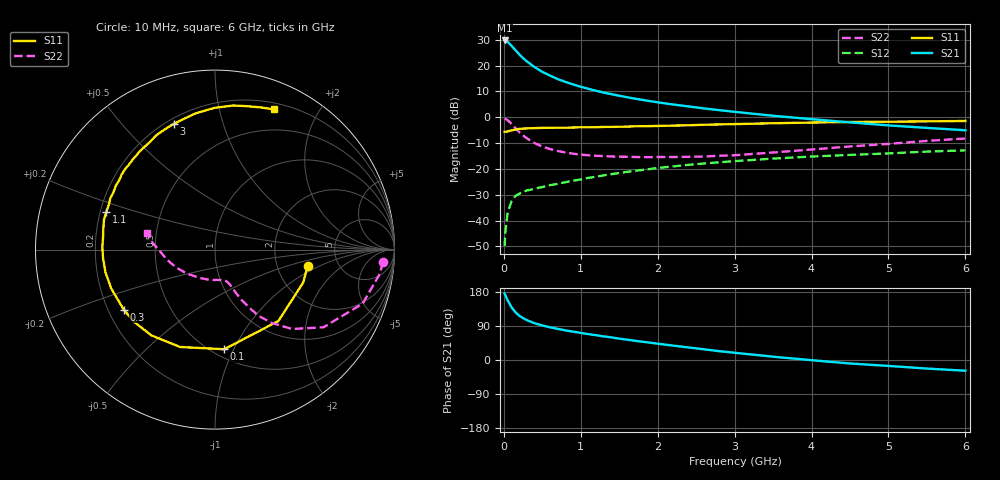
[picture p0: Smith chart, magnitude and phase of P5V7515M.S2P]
! SIEMENS Small Signal Semiconductors
! BFP183
! Si NPN RF Bipolar Junction Transistor in SOT143
! VCE = 0.75 V  IC = 15 mA
! Common Emitter S-Parameters:  March  1996
# GHz  S  MA  R  50
!  f  S11  S21  S12  S22
! GHz  MAG  ANG  MAG  ANG  MAG  ANG  MAG  ANG
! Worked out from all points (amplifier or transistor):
!   36 points, 10 MHz to 6 GHz, reference 50 ohm
!   highest |S21| = 29.7 dB at 10 MHz (marker M1)
!   |S21| within 3 dB of that: start of sweep to 127.7 MHz
!   unconditionally stable (mu >= 1): 673.4 MHz to end of sweep
!   at 250 MHz: K = 0.50, MSG = 25.9 dB, |S12| = -28.9 dB
!   at 1.4 GHz: K = 1.28, MAG = 12.3 dB, |S12| = -22.0 dB
!   at 6 GHz: K = 1.10, MAG = 2.0 dB, |S12| = -12.8 dB
!   S11 on the Smith chart (normalised r, x): 10 MHz: 2.99, -0.76; 100 MHz: 0.57, -0.92; 300 MHz: 0.26, -0.28; 1.1 GHz: 0.22, +0.16; 3 GHz: 0.23, +0.70; 6 GHz: 0.27, +1.47
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0.01  0.524 -10.1  30.66 175.4  0.0032 80.0  0.9386 -4.2
0.02  0.5247 -20.4  30.5 170.8  0.0061 82.2  0.928 -8.4
0.05  0.532 -48.4  28.9 157.1  0.0144 73.6  0.8759 -20.1
0.1  0.5574 -84.7  24.16 139.3  0.0237 57.5  0.7435 -35.6
0.15  0.5764 -109.7  19.92 126.1  0.0299 49.9  0.617 -45.8
0.2  0.5949 -126.5  16.56 117.0  0.0332 44.2  0.5176 -52.2
0.25  0.6041 -138.0  13.96 110.4  0.0359 41.9  0.4458 -56.4
0.3  0.6086 -146.7  12.04 105.2  0.0383 41.5  0.3904 -58.8
0.4  0.6176 -159.6  9.326 97.0  0.0413 40.3  0.3157 -62.3
0.5  0.6232 -168.3  7.559 91.2  0.0448 40.3  0.2708 -64.1
0.6  0.6256 -175.5  6.414 86.3  0.0486 42.1  0.2427 -65.3
0.7  0.6279 178.6  5.479 82.1  0.0514 43.3  0.2222 -66.2
0.8  0.6275 173.7  4.839 78.2  0.0553 44.2  0.2082 -67.2
1.1  0.6404 161.1  3.553 68.2  0.0673 46.2  0.1837 -71.4
1.3  0.6496 154.0  2.998 62.2  0.0751 46.3  0.1773 -75.0
1.6  0.6596 143.9  2.448 53.7  0.0876 46.2  0.1719 -81.1
2.2  0.6895 127.3  1.765 38.0  0.112 42.9  0.1698 -98.1
3  0.7373 108.1  1.274 19.1  0.1416 36.4  0.1841 -124.7
3.5  0.7659 98.4  1.069 8.7  0.1586 32.0  0.208 -140.8
4.5  0.8092 82.8  0.797 -9.2  0.1868 22.9  0.2723 -167.7
5.5  0.8332 71.8  0.623 -22.6  0.2166 14.8  0.3489 174.0
6  0.8477 67.1  0.561 -28.3  0.2289 10.1  0.3887 166.2
